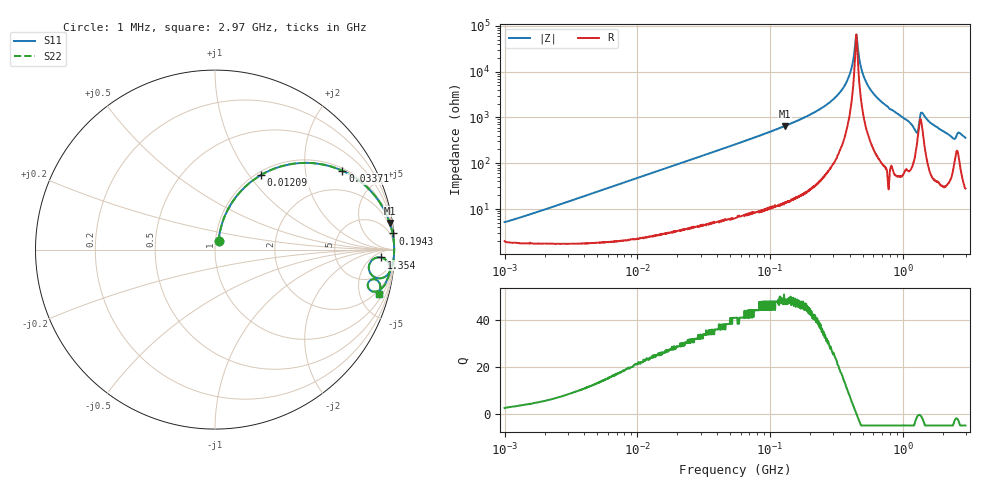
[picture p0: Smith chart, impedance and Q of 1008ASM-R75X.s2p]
!s-Parameter Generated by FASTRON Sdn. Bhd.
!FASTRON P/N : 1008ASM-R75X
!Keysight Technologies: E4991B_MY54100416_A.01.15
!Date: Tue Nov 21 09:33:54 2023
!Version  :Rev00  Wed Nov 22 15:17:14 2023
!Data & Calibration Information:
!Freq  S11  S21  S12  S22
!PortZ  Port1:50+j0  Port2:50+j0
!When reading reference impedance value at option line is always used.
! Remarks : This data is being provided solely for informational purposes.
# Hz S dB R 50
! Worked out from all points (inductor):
!   1599 points, 1 MHz to 2.97 GHz, reference 50 ohm
!   read as one part in series: L = 763 nH near 1.145 MHz
!   highest Q = 48.5 at 130.2 MHz (marker M1), where L = 796 nH
!   self-resonance near 445.8 MHz
!   S11 on the Smith chart (normalised r, x): 1 MHz: 1.04, +0.10; 12.09 MHz: 1.05, +1.15; 33.71 MHz: 1.10, +3.17; 194.3 MHz: 1, +22; 1.354 GHz: 19, -12; 2.97 GHz: 1.56, -7.16
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1000000  -25.90 64.7  -0.18 -2.7  -0.18 -2.7  -25.90 64.7
3804036  -15.10 74.3  -0.29 -10.1  -0.29 -10.1  -15.10 74.3
1.20852e7  -6.21 58.3  -1.40 -29.2  -1.40 -29.2  -6.21 58.3
1.439846e7  -5.13 54.1  -1.82 -33.6  -1.82 -33.6  -5.13 54.1
3.371011e7  -1.57 31.7  -5.57 -56.6  -5.57 -56.6  -1.57 31.7
5.477226e7  -0.68 21.0  -8.92 -67.6  -8.92 -67.6  -0.68 21.0
1.30174e8  -0.13 8.7  -16.40 -80.1  -16.40 -80.1  -0.13 8.7
1.942587e8  -0.05 5.2  -20.90 -83.5  -20.90 -83.5  -0.05 5.2
2.073156e8  -0.05 4.7  -21.70 -83.9  -21.70 -83.9  -0.05 4.7
2.884452e8  -0.02 2.5  -27.10 -85.4  -27.10 -85.4  -0.02 2.5
3.594878e8  -0.02 1.2  -33.20 -84.8  -33.20 -84.8  -0.02 1.2
4.0536e8  -0.01 0.6  -40.00 -80.6  -40.00 -80.6  -0.01 0.6
4.480278e8  -0.01 -0.0  -56.20 1.9  -56.20 1.9  -0.01 -0.0
4.902556e8  -0.01 -0.5  -40.80 79.2  -40.80 79.2  -0.01 -0.5
5.337858e8  -0.02 -1.0  -35.10 83.5  -35.10 83.5  -0.02 -1.0
7.846996e8  -0.03 -3.5  -24.20 85.5  -24.20 85.5  -0.03 -3.5
1.255985e9  -0.74 -10.0  -14.60 58.9  -14.60 58.9  -0.74 -10.0
1.353887e9  -0.67 -2.7  -21.20 30.1  -21.20 30.1  -0.67 -2.7
1.409185e9  -0.32 -4.0  -22.20 60.0  -22.20 60.0  -0.32 -4.0
2.371269e9  -0.68 -14.7  -11.80 65.9  -11.80 65.9  -0.68 -14.7
2.647227e9  -0.68 -10.9  -14.10 62.4  -14.10 62.4  -0.68 -10.9
2.970126e9  -0.50 -15.2  -11.60 70.3  -11.60 70.3  -0.50 -15.2
